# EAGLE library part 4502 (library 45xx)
Stored hex INVERTER/BUFFER
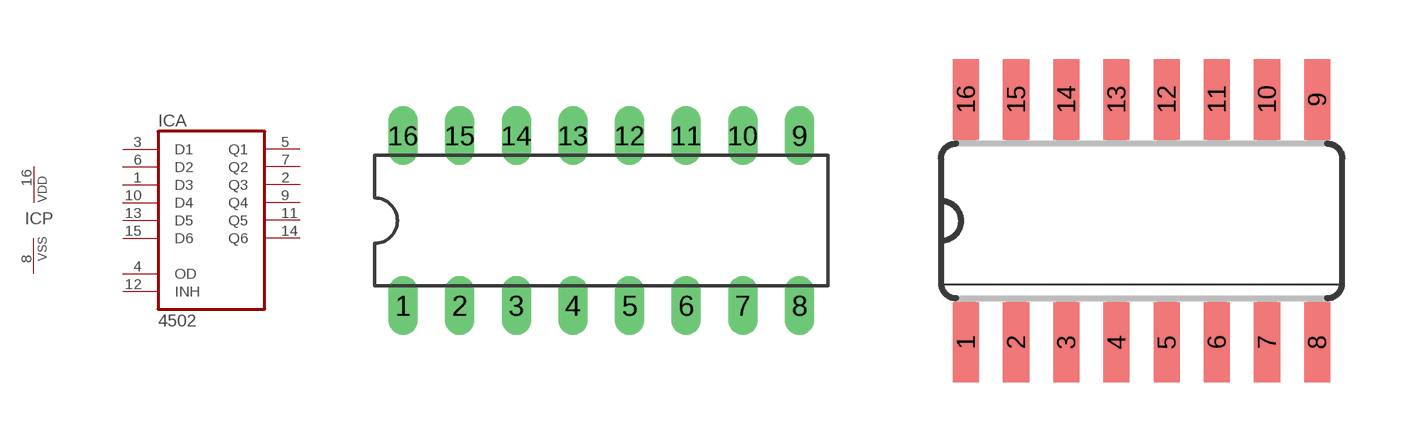
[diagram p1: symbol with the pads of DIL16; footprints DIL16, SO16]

Designator prefix IC; gates A=4502 P=PWRN

## 4502N  [DIL16]
1  A:D3  in
2  A:Q3  out
3  A:D1  in
4  A:OD  in
5  A:Q1  out
6  A:D2  in
7  A:Q2  out
8  P:VSS  pwr
9  A:Q4  out
10  A:D4  in
11  A:Q5  out
12  A:INH  in
13  A:D5  in
14  A:Q6  out
15  A:D6  in
16  P:VDD  pwr

## 4502D  [SO16]
Pads as for DIL16

## Footprint DIL16 (pad centres in mm)
Dual In Line Package
drill 0.813 long: 1 -8.89,-3.81; 2 -6.35,-3.81; 3 -3.81,-3.81; 4 -1.27,-3.81; 5 1.27,-3.81; 6 3.81,-3.81; 7 6.35,-3.81; 8 8.89,-3.81; 9 8.89,3.81; 10 6.35,3.81; 11 3.81,3.81; 12 1.27,3.81; 13 -1.27,3.81; 14 -3.81,3.81; 15 -6.35,3.81; 16 -8.89,3.81

## Footprint SO16 (pad centres in mm)
Small Outline package 150 mil
smd 0.66 x 2.032: 1 -4.445,-3.073; 2 -3.175,-3.073; 3 -1.905,-3.073; 4 -0.635,-3.073; 5 0.635,-3.073; 6 1.905,-3.073; 7 3.175,-3.073; 8 4.445,-3.073; 9 4.445,3.073; 10 3.175,3.073; 11 1.905,3.073; 12 0.635,3.073; 13 -0.635,3.073; 14 -1.905,3.073; 15 -3.175,3.073; 16 -4.445,3.073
